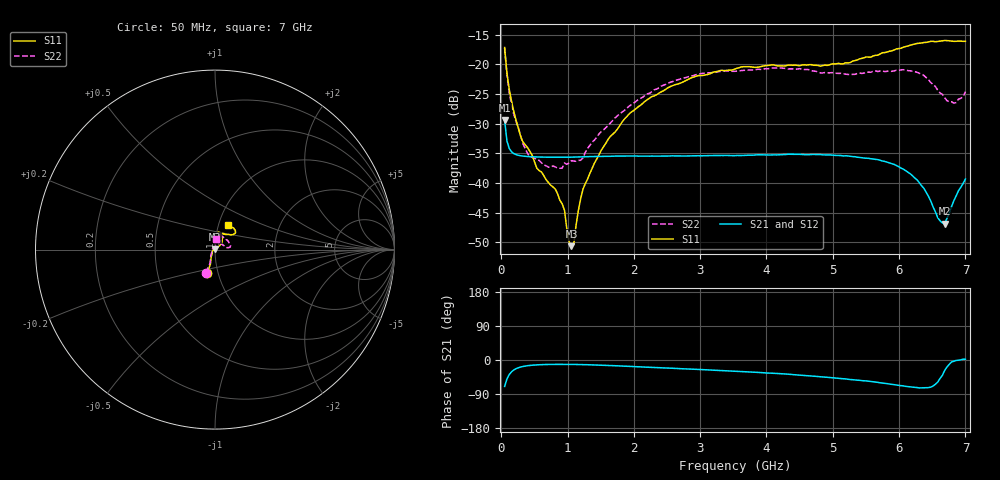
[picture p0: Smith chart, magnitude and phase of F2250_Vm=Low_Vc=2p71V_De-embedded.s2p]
! Integrated Device Technology
! Corporate Headquarters
! 6024 Silver Creek Valley Road
! San Jose, CA 95138  USA
! Phone:  1-408-284-8200
! Toll Free:  1-800-223-1366
! Webpage:  http://www.idt.com/
! Timing and RF Division
! 515 Groton Road, Suite 102
! Westford, MA 01886-6024
! Device:  F2250
! Description: Voltage Variable RF Attenuator
! Frequency:  50.0 -  6000.00 MHz
! Package:  3x3 mm Thin QFN Plastic Package: 16 pin
! Ports:  2 RF, 3 DC
!  Pin  1  = GND
!  Pin  2  = NC
!  Pin  3  = RF1  = Port 1
!  Pin  4  = NC
!  Pin  5  = GND
!  Pin  6  = GND
!  Pin  7  = GND
!  Pin  8  = GND
!  Pin  9  = NC
!  Pin 10  = RF2  = Port 2
!  Pin 11  = NC
!  Pin 12  = GND
!  Pin 13  = GND
!  Pin 14  = VCNTRL
!  Pin 15  = VDD
!  Pin 16  = VMODE
! Vcntrl:  2.710 Volts
! Vmode:  +0.000 Volts
! Vdd:  +3.30  Volts
! Current:  1.176 mA
! Data:  The device was measured on a the F2250 evaluation board which has
!  individual transmission lines to the RF pins.  Data was collected
!  using a calibrated network analyzer.  The evaluation board was
!  de-embedded using a TRL calibration technique.
!  The reference plane is the edge of the package pin.
! Misc:  SN 10
!  Action Tracker AT0258
! Date Measured:  2014-11-26
! Date:  2015-10-15  MJV
! Note:
!  Integrated Device Technology supplies this data as a sample of measured
!  data at the package pin for this product.  Your particular data for this
!  product may vary.
!  Data was taken at 25 degrees C.
!  Integrated Device Technology reserves the right to change this data at anytime.
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# GHz S dB R 50
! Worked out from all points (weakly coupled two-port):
!   201 points, 50 MHz to 7 GHz, reference 50 ohm
!   highest |S21| = -29.41 dB at 50 MHz (marker M1); lowest = -46.9 dB at 6.687 GHz (marker M2)
!   lowest |S11| = -50.7 dB at 1.058 GHz (marker M3), VSWR 1.01, Z = 49.8 + j0.243 ohm
!   |S11| at or under -10 dB: start of sweep to end of sweep
!   |S22| runs from -37.5 to -17.3 dB; largest |S21 - S12| = 5.6e-05
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0.05  -17.18 -108.6  -29.41 -69.8  -29.42 -69.8  -17.28 -111.0
0.08475  -21.45 -107.5  -32.92 -50.4  -32.92 -50.3  -21.74 -110.2
0.15425  -26.23 -116.6  -34.76 -31.2  -34.75 -31.2  -26.81 -122.5
0.29325  -32.21 -127.9  -35.43 -18.5  -35.43 -18.5  -32.09 -137.4
0.3975  -34.09 -141.8  -35.56 -15.0  -35.56 -15.0  -35.06 -160.4
0.91875  -43.54 157.7  -35.68 -11.5  -35.68 -11.5  -37.51 133.5
0.9535  -44.63 169.9  -35.68 -11.5  -35.68 -11.5  -36.65 131.1
1.023  -49.91 143.8  -35.68 -11.6  -35.67 -11.6  -36.64 115.9
1.05775  -50.67 123.7  -35.67 -11.6  -35.67 -11.6  -36.27 110.7
1.0925  -50.45 89.6  -35.66 -11.7  -35.66 -11.7  -36.31 106.4
1.162  -44.69 56.8  -35.64 -11.9  -35.64 -11.9  -36.21 95.4
1.2315  -41.10 44.5  -35.61 -12.1  -35.61 -12.1  -35.79 85.8
1.6485  -32.11 42.0  -35.52 -14.6  -35.52 -14.6  -29.88 64.6
1.9265  -28.40 41.3  -35.47 -16.9  -35.46 -16.9  -27.09 56.7
2.37825  -24.87 47.3  -35.48 -20.3  -35.48 -20.3  -23.99 56.8
3.525  -20.80 72.5  -35.41 -29.5  -35.40 -29.6  -21.19 74.7
4.7065  -20.17 72.3  -35.20 -42.6  -35.20 -42.6  -21.15 72.3
5.85325  -17.81 40.4  -36.64 -63.3  -36.64 -63.3  -21.13 23.0
6.27025  -16.50 40.0  -39.49 -72.6  -39.50 -72.7  -21.36 9.6
6.68725  -15.99 48.8  -46.87 -27.7  -46.85 -27.4  -25.64 28.5
6.861  -16.13 55.1  -42.19 -1.3  -42.14 -1.3  -26.46 58.0
7  -16.13 63.2  -39.35 1.9  -39.31 1.7  -24.62 83.1
